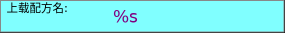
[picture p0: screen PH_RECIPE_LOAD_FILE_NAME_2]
VISUALIZATION PH_RECIPE_LOAD_FILE_NAME_2  // 285x33
VAR_IN_OUT
	RECIPE_CTRL_V2 : ST_RecipeCtrl_2;
END_VAR
VAR_INPUT
	Right_Edge_Rel : UDINT;
END_VAR
    Rectangle (0,0 285x33), "上载配方名:", input disabled if: true, text list: 'TextList_Recipe', text index: 103
        p874137650: Right_Edge_Rel
    Rectangle (110,0 175x33), "%s", text variable: RECIPE_CTRL_V2.sgFileNameLoad
        p874137650: Right_Edge_Rel
        OnMouseClick: write the text variable via Edit
END_VISUALIZATION
